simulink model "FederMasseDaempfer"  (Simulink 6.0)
settings: Solver=ode45  StartTime=0.0  StopTime=100.0  FixedStep=0.01  RelTol=1e-6
libraries: simulink x1

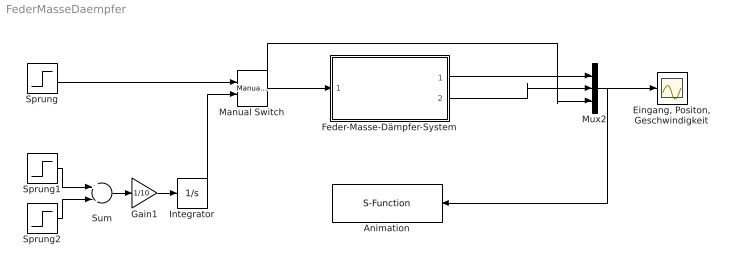
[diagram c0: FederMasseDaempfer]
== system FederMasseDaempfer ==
  Animation : S-Function  Orientation=left  FunctionName=FMDAnim  Parameters=T  mask{T=0.1}
      mask prompts: T "Animationsintervall"
  "Eingang, Positon, Geschwindigkeit" : Scope
  Feder-Masse-Dämpfer-System : Subsystem  mask{D=0.1, w0=0.5}
      mask prompts: D "Dämpfung"; w0 "Eigenkreisfrequenz"
  Gain1 : Gain  Gain=1/10  ParameterDataType=sfix(16)  ParameterScaling=2^0  OutDataType=sfix(16)  OutScaling=2^0
  Integrator : Integrator
  Manual Switch : simulink/Signal Routing/Manual Switch  SystemSampleTime=-1  sw=0  action=0
  Mux2 : Mux  Inputs=3
  Sprung : Step  Time=5  SampleTime=0
  Sprung1 : Step  Time=5  SampleTime=0
  Sprung2 : Step  Time=15  SampleTime=0
  Sum : Sum  Inputs=+-  OutDataType=sfix(16)  OutScaling=2^0
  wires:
  Manual Switch/1 -> Mux2/3, Feder-Masse-Dämpfer-System/1(Eingang)
  Mux2/1 -> "Eingang, Positon, Geschwindigkeit"/1, Animation/1
  Feder-Masse-Dämpfer-System/1(Position) -> Mux2/1
  Feder-Masse-Dämpfer-System/2(Geschwindigkeit) -> Mux2/2
  Sprung/1 -> Manual Switch/1
  Sprung1/1 -> Sum/1
  Sum/1 -> Gain1/1
  Gain1/1 -> Integrator/1
  Sprung2/1 -> Sum/2
  Integrator/1 -> Manual Switch/2

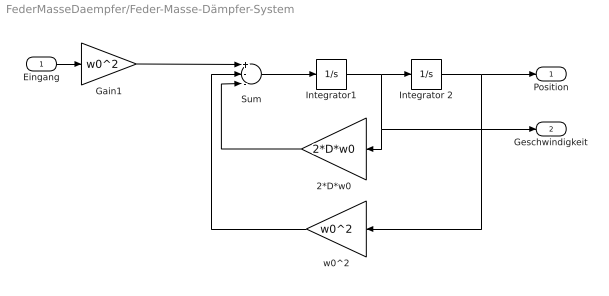
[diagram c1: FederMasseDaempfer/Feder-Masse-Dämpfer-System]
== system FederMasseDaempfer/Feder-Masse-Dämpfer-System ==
  Eingang : Inport  OutDataType=sfix(16)  OutScaling=2^0
  2*D*w0 : Gain  Orientation=left  Gain=2*D*w0  ParameterDataType=sfix(16)  ParameterScaling=2^0  OutDataType=sfix(16)  OutScaling=2^0
  Gain1 : Gain  Gain=w0^2  ParameterDataType=sfix(16)  ParameterScaling=2^0  OutDataType=sfix(16)  OutScaling=2^0
  Integrator 2 : Integrator
  Integrator1 : Integrator
  Sum : Sum  Inputs=+--  OutDataType=sfix(16)  OutScaling=2^0
  w0^2 : Gain  Orientation=left  Gain=w0^2  ParameterDataType=sfix(16)  ParameterScaling=2^0  OutDataType=sfix(16)  OutScaling=2^0
  Position : Outport  OutDataType=sfix(16)  OutScaling=2^0
  Geschwindigkeit : Outport  Port=2  OutDataType=sfix(16)  OutScaling=2^0
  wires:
  Eingang/1 -> Gain1/1
  w0^2/1 -> Sum/2
  2*D*w0/1 -> Sum/3
  Integrator 2/1 -> Position/1, w0^2/1
  Gain1/1 -> Sum/1
  Integrator1/1 -> Integrator 2/1, 2*D*w0/1, Geschwindigkeit/1
  Sum/1 -> Integrator1/1
